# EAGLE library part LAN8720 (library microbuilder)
LAN8720A 10/100 Ethernet PHY Mouser: 886-LAN8720AI-CP
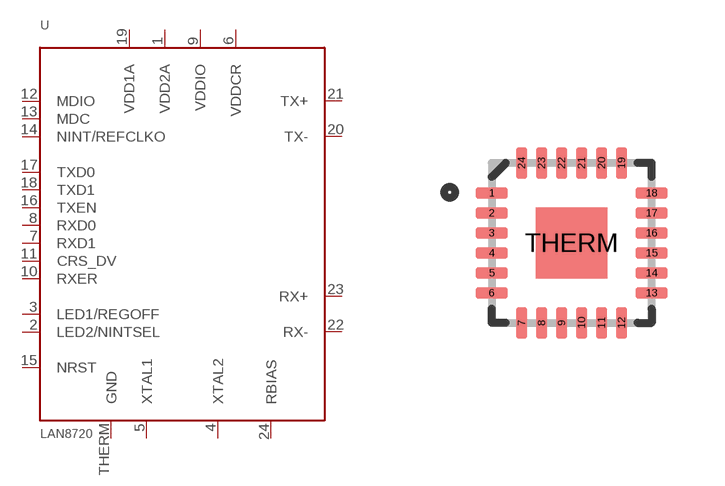
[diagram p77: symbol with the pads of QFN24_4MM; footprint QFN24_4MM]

Designator prefix U

## LAN8720  [QFN24_4MM]
1  VDD2A
2  LED2/NINTSEL
3  LED1/REGOFF
4  XTAL2
5  XTAL1
6  VDDCR
7  RXD1
8  RXD0
9  VDDIO
10  RXER
11  CRS_DV
12  MDIO
13  MDC
14  NINT/REFCLKO
15  NRST
16  TXEN
17  TXD0
18  TXD1
19  VDD1A
20  TX-
21  TX+
22  RX-
23  RX+
24  RBIAS
THERM  GND

## Footprint QFN24_4MM (pad centres in mm)
smd 0.8 x 0.28: 1 -2,1.25; 2 -2,0.75; 3 -2,0.25; 4 -2,-0.25; 5 -2,-0.75; 6 -2,-1.25; 13 2,-1.25; 14 2,-0.75; 15 2,-0.25; 16 2,0.25; 17 2,0.75; 18 2,1.25
smd 0.28 x 0.8: 7 -1.25,-2; 8 -0.75,-2; 9 -0.25,-2; 10 0.25,-2; 11 0.75,-2; 12 1.25,-2; 19 1.25,2; 20 0.75,2; 21 0.25,2; 22 -0.25,2; 23 -0.75,2; 24 -1.25,2
smd 1.778 x 1.778: THERM 0,0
